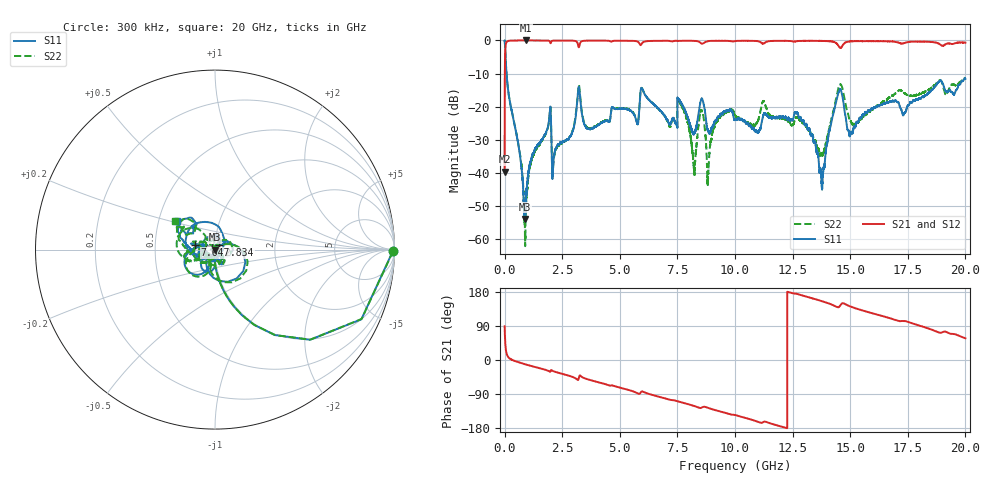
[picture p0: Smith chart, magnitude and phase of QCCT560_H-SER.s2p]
!{QCCT560}
!Johanson Technology Inc.
!www.johansontechnology.com
!Test Board Conditions:
!Substrate Type  RO4350B
!Substrate Thickness  20 mil
!Substrate Dk  3.66
!TL Type: GCPW
!TL Trace Width  34 mil
!TL Gap  10 mil
!Electrode orientation  Horizontal
!DUT TOPOLOGY	SERIES
!Mounting Pad LxW  26x52 mil
! Created Sat Jan  9 19:19:56 2021
# hz S ma R 50
! 2 Port Network Data from SP1.SP block
! freq  magS11  angS11  magS21  angS21  magS12  angS12  magS22  angS22
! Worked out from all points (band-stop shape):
!   20001 points, 300 kHz to 20 GHz, reference 50 ohm
!   highest |S21| = 0.00 dB at 936.3 MHz (marker M1); lowest = -39.6 dB at 300 kHz (marker M2)
!   |S21| within 3 dB of the highest: 28.26 MHz to end of sweep
!   lowest |S11| = -53.8 dB at 866.3 MHz (marker M3), VSWR 1.00, Z = 49.8 - j0.0681 ohm
!   |S11| at or under -10 dB: 83.89 MHz to end of sweep
!   |S22| runs from -62.0 to 0.0 dB; largest |S21 - S12| = 0.016
!   S11 on the Smith chart (normalised r, x): 300 kHz: open; 2.834 GHz: 1.05, +0.06; 7.647 GHz: 0.80, +0.04; 20 GHz: 0.62, +0.21
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300000  0.9905 -0.5  0.01052 88.9  0.01062 89.6  0.9915 -0.6
1.193e8  0.2271 -78.5  0.973 11.5  0.9734 11.5  0.2281 -78.4
8.663e8  0.002034 -160.4  0.9997 -10.9  0.9988 -10.9  0.002142 -76.9
9.363e8  0.004502 101.0  0.9999 -12.1  0.9988 -12.1  0.003789 57.1
1.1613e9  0.01644 82.3  0.9991 -15.9  0.9992 -15.8  0.01542 66.6
1.9183e9  0.05877 51.0  0.9906 -29.2  0.99 -29.2  0.05789 57.4
2.1363e9  0.01735 51.8  0.9959 -30.1  0.9958 -30.1  0.01633 53.8
2.8343e9  0.03526 49.5  0.9946 -42.3  0.9954 -42.3  0.03556 41.0
3.3343e9  0.0882 -123.5  0.9666 -43.8  0.9671 -43.8  0.09324 -109.8
6.6673e9  0.09518 170.5  0.9883 -96.5  0.9883 -96.4  0.09394 179.5
7.6473e9  0.1155 166.9  0.9863 -111.2  0.9862 -111.2  0.1084 154.6
8.2233e9  0.03893 -129.8  0.9855 -121.3  0.9859 -121.2  0.01093 68.2
8.5343e9  0.1296 -107.3  0.9032 -126.3  0.9024 -126.3  0.08854 -86.5
8.8403e9  0.04258 -118.1  0.9771 -126.4  0.9769 -126.5  0.009694 -56.9
9.2283e9  0.06794 -67.3  0.987 -133.7  0.9865 -133.8  0.06031 -39.2
1.00003e10  0.06372 -65.9  0.9757 -145.1  0.9771 -145.1  0.07295 -74.6
1.33343e10  0.03865 54.1  0.9865 163.1  0.9872 163.1  0.03669 99.0
1.37573e10  0.006966 -8.4  0.9854 155.6  0.984 155.6  0.0193 147.9
1.45303e10  0.1765 154.6  0.7889 140.7  0.7918 140.6  0.2097 179.6
1.50203e10  0.04008 -42.7  0.9666 141.0  0.9696 140.9  0.06117 145.3
1.66673e10  0.1157 -161.3  0.9707 111.1  0.9628 111.2  0.1361 -152.4
2e10  0.2648 143.1  0.9243 57.2  0.9158 57.1  0.276 144.6
